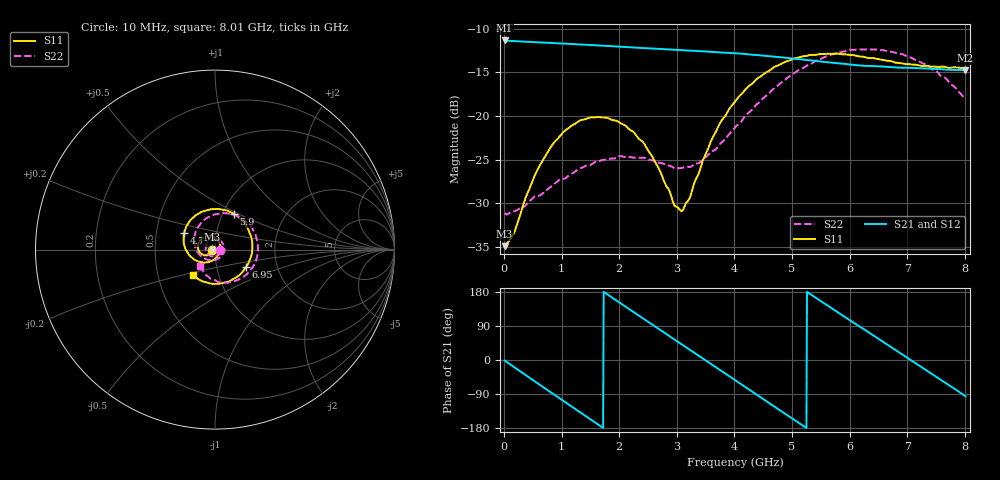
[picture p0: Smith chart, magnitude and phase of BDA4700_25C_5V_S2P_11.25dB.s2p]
!Agilent Technologies,E5071B,MY42404982,A.09.10
!Date: Mon Oct 20 13:31:43 2025
!Data & Calibration Information:
!Freq	S11:SOLT2(ON)	S21:SOLT2(ON)	S12:SOLT2(ON)	S22:SOLT2(ON)
# Hz S RI R 50
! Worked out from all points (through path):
!   801 points, 10 MHz to 8.01 GHz, reference 50 ohm
!   highest |S21| = -11.36 dB at 10 MHz (marker M1); lowest = -14.8 dB at 8.01 GHz (marker M2)
!   group delay of S21, straight-line fit = 282 ps
!   lowest |S11| = -34.9 dB at 10 MHz (marker M3), VSWR 1.04, Z = 48.2 - j0.105 ohm
!   |S11| at or under -10 dB: start of sweep to end of sweep
!   |S22| runs from -31.3 to -12.4 dB; largest |S21 - S12| = 0.002
!   S11 on the Smith chart (normalised r, x): 10 MHz: 0.96, -0.00; 4.77 GHz: 0.70, +0.14; 5.9 GHz: 1.13, +0.47; 6.95 GHz: 1.38, -0.28; 8.01 GHz: 0.75, -0.22
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1e7  -0.018 -0.00109  0.2702 -0.0059  0.2701 -0.00622  0.0277 -0.00148
1.6e8  -0.0188 -0.00937  0.256 -0.0792  0.2559 -0.0792  0.0268 -0.00927
5.1e8  -0.0336 -0.028  0.156 -0.2137  0.156 -0.2137  0.0142 -0.0311
7.2e8  -0.0497 -0.0321  0.0646 -0.2544  0.0646 -0.2544  -0.00189 -0.0371
1.02e9  -0.0768 -0.0229  -0.0752 -0.2483  -0.0753 -0.2483  -0.0286 -0.033
1.35e9  -0.0948 0.0065  -0.199 -0.1611  -0.1992 -0.1613  -0.0501 -0.00614
1.94e9  -0.0658 0.0672  -0.2319 0.0928  -0.232 0.0929  -0.0251 0.0515
2.41e9  -0.00798 0.0704  -0.084 0.2296  -0.084 0.2299  0.0284 0.0503
2.68e9  0.0185 0.0469  0.0311 0.2401  0.0311 0.2399  0.0482 0.0242
2.96e9  0.0292 0.00947  0.14 0.1935  0.1402 0.1933  0.0495 -0.0093
3.1e9  0.0267 -0.0107  0.1829 0.152  0.1824 0.1525  0.043 -0.0267
3.54e9  -0.0171 -0.0623  0.2326 -0.0202  0.2326 -0.0205  -0.00677 -0.0593
4.01e9  -0.1041 -0.0609  0.1376 -0.1822  0.1377 -0.182  -0.0771 -0.0375
4.39e9  -0.1631 -0.00081  -0.00693 -0.2229  -0.00691 -0.2233  -0.114 0.0252
4.77e9  -0.1709 0.0939  -0.1415 -0.1646  -0.1409 -0.1652  -0.1031 0.1105
5.35e9  -0.0647 0.2138  -0.2046 0.0343  -0.2047 0.0337  0.0198 0.1993
5.9e9  0.1042 0.1994  -0.0847 0.1796  -0.085 0.1794  0.177 0.1524
6.3e9  0.1875 0.1058  0.0465 0.1877  0.0476 0.1868  0.2372 0.0394
6.68e9  0.2058 -0.0181  0.15 0.1174  0.1504 0.1174  0.2206 -0.0771
6.95e9  0.1723 -0.0983  0.185 0.0375  0.1852 0.0366  0.1714 -0.1424
7.48e9  0.0315 -0.1888  0.1384 -0.1242  0.1385 -0.1246  0.0225 -0.1819
8.01e9  -0.123 -0.143  -0.0174 -0.1818  -0.0171 -0.182  -0.0826 -0.0932
